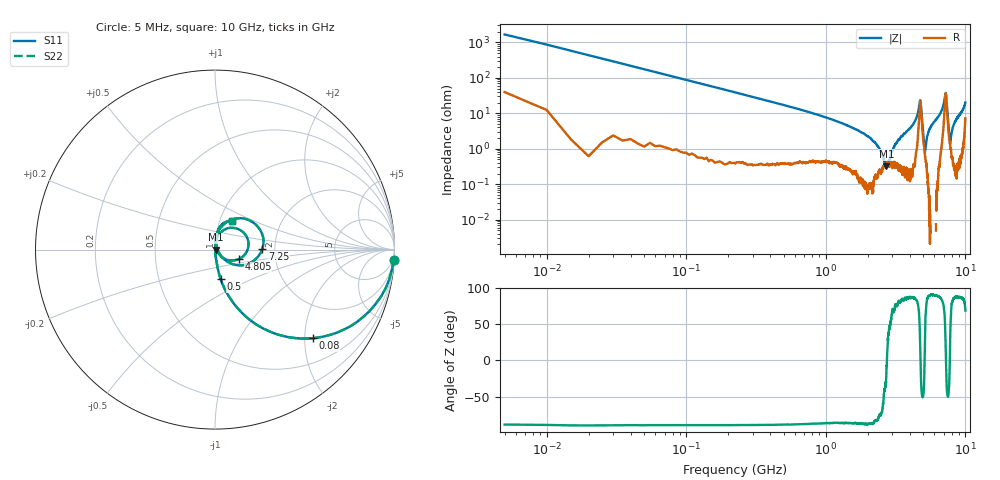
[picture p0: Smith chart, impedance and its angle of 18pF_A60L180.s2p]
! Amotech Co.,Ltd.
! http://www.amotech.co.kr/
! Part Number: A60L180
! These Parameters are Measured in Series Mode Connection
! Operation Temp=25[degC], DC Bias Voltage=0[V]
! Freq. Start=5[MHz] Stop=10[GHz], 2000[Steps]
! Date: Monday, July 14, 2020, 09:36:59
# GHZ S RI R 50.000000
!Freq.(Hz) S11(Real) S11(Imag) S21(Real) S21(Imag) S12(Real) S12(Imag) S22(Real) S22(Imag)
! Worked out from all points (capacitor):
!   2000 points, 5 MHz to 10 GHz, reference 50 ohm
!   read as one part in series: C = 18.2 pF near 55 MHz
!   lowest |Z| = 320 mohm at 2.72 GHz (marker M1)
!   series resonance near 2.738 GHz, so ESL is about 190 pH
!   S11 on the Smith chart (normalised r, x): 5 MHz: 2, -33; 80 MHz: 1.02, -2.19; 500 MHz: 1.01, -0.34; 4.805 GHz: 1.29, -0.14; 7.25 GHz: 1.72, +0.02; 10 GHz: 1.15, +0.38
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0.005  0.995 -0.0593  0.00495 0.0593  0.00495 0.0593  0.995 -0.0593
0.08  0.545 -0.4938  0.455 0.4938  0.455 0.4938  0.545 -0.4938
0.21  0.1502 -0.3525  0.8498 0.3525  0.8498 0.3525  0.1502 -0.3525
0.5  0.0321 -0.1652  0.9679 0.1652  0.9679 0.1652  0.0321 -0.1652
1.675  0.0031 -0.0339  0.9969 0.0339  0.9969 0.0339  0.0031 -0.0339
2.28  0.0021 -0.0139  0.9979 0.0139  0.9979 0.0139  0.0021 -0.0139
2.72  0.00309 -0.000784  0.9969 0.000784  0.9969 0.000784  0.00309 -0.000784
3.34  0.00311 0.0182  0.9969 -0.0182  0.9969 -0.0182  0.00311 0.0182
4.36  0.00761 0.0594  0.9924 -0.0594  0.9924 -0.0594  0.00761 0.0594
4.725  0.1653 0.088  0.8347 -0.088  0.8347 -0.088  0.1653 0.088
4.805  0.1317 -0.0533  0.8683 0.0533  0.8683 0.0533  0.1317 -0.0533
5.005  0.0156 -0.0163  0.9844 0.0163  0.9844 0.0163  0.0156 -0.0163
5.14  0.00635 0.00474  0.9937 -0.00474  0.9937 -0.00474  0.00635 0.00474
5.31  0.00245 0.0211  0.9975 -0.0211  0.9975 -0.0211  0.00245 0.0211
5.505  0.00167 0.0345  0.9983 -0.0345  0.9983 -0.0345  0.00167 0.0345
6.67  0.0187 0.1031  0.9813 -0.1031  0.9813 -0.1031  0.0187 0.1031
7.105  0.1477 0.1744  0.8523 -0.1744  0.8523 -0.1744  0.1477 0.1744
7.25  0.2643 0.00534  0.7357 -0.00534  0.7357 -0.00534  0.2643 0.00534
7.36  0.132 -0.088  0.868 0.088  0.868 0.088  0.132 -0.088
7.76  0.013 0.00419  0.987 -0.00419  0.987 -0.00419  0.013 0.00419
8.335  0.00523 0.0523  0.9948 -0.0523  0.9948 -0.0523  0.00523 0.0523
10  0.0957 0.1591  0.9043 -0.1591  0.9043 -0.1591  0.0957 0.1591
